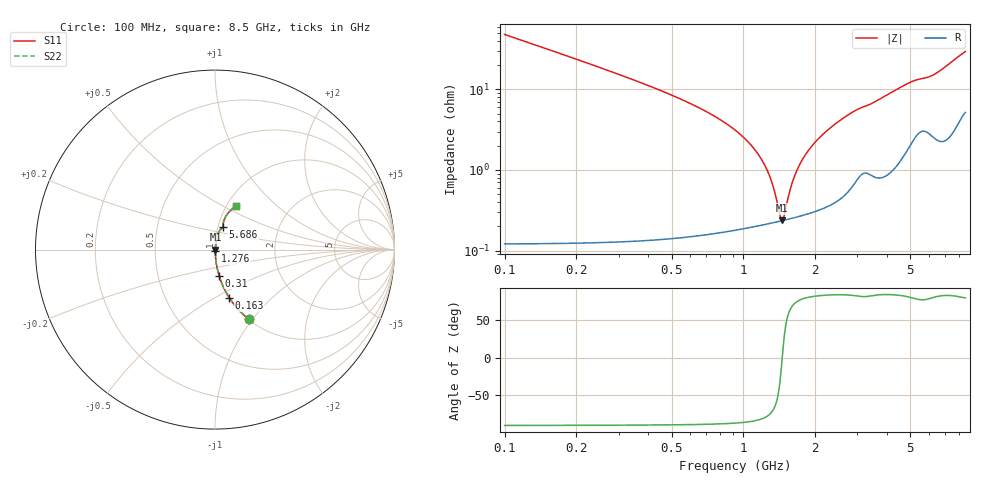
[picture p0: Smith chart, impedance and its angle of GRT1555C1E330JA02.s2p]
!Murata Part Number: GRT1555C1E330JA02
!These Parameters are Measured in Series Mode Connection
!Data Generated on Jun 19, 2026
!  o--ll--o
!Port1  Port2
!  o------o
!Operation Temp=25[degC], DC Bias Voltage=0[V]
!Freq. Start=100[MHz] Stop=9[GHz] 401[Steps]
# Hz S RI R 50
!Freq.(Hz) S11(Real) S11(Imag) S21(Real) S21(Imag) S12(Real) S12(Imag) S22(Real) S22(Imag)
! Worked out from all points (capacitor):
!   401 points, 100 MHz to 8.5 GHz, reference 50 ohm
!   read as one part in series: C = 33 pF near 142 MHz
!   lowest |Z| = 238 mohm at 1.444 GHz (marker M1)
!   series resonance near 1.454 GHz, so ESL is about 360 pH
!   S11 on the Smith chart (normalised r, x): 100 MHz: 1.00, -0.96; 163 MHz: 1.00, -0.58; 310 MHz: 1.00, -0.30; 1.276 GHz: 1.00, -0.02; 5.686 GHz: 1.06, +0.27; 8.5 GHz: 1.10, +0.58
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1e8  0.1879 -0.3893  0.8121 0.3893  0.8121 0.3893  0.1879 -0.3893
1.63e8  0.0796 -0.2686  0.9204 0.2686  0.9204 0.2686  0.0796 -0.2686
3.1e8  0.0228 -0.1449  0.9772 0.1449  0.9772 0.1449  0.0228 -0.1449
5.62e8  0.00672 -0.0724  0.9933 0.0724  0.9933 0.0724  0.00672 -0.0724
1.024e9  0.00245 -0.0237  0.9976 0.0237  0.9976 0.0237  0.00245 -0.0237
1.171e9  0.00225 -0.0144  0.9978 0.0144  0.9978 0.0144  0.00225 -0.0144
1.276e9  0.00222 -0.00867  0.9978 0.00867  0.9978 0.00867  0.00222 -0.00867
1.402e9  0.00229 -0.0024  0.9977 0.0024  0.9977 0.0024  0.00229 -0.0024
1.444e9  0.00233 -0.000437  0.9977 0.000437  0.9977 0.000437  0.00233 -0.000437
1.465e9  0.00236 0.000524  0.9976 -0.000524  0.9976 -0.000524  0.00236 0.000524
1.507e9  0.00241 0.00241  0.9976 -0.00241  0.9976 -0.00241  0.00241 0.00241
1.57e9  0.0025 0.00515  0.9975 -0.00515  0.9975 -0.00515  0.0025 0.00515
1.654e9  0.00265 0.00866  0.9973 -0.00866  0.9973 -0.00866  0.00265 0.00866
1.759e9  0.00287 0.0129  0.9971 -0.0129  0.9971 -0.0129  0.00287 0.0129
1.906e9  0.00325 0.0185  0.9968 -0.0185  0.9968 -0.0185  0.00325 0.0185
2.305e9  0.00469 0.0326  0.9953 -0.0326  0.9953 -0.0326  0.00469 0.0326
2.914e9  0.00948 0.0525  0.9905 -0.0525  0.9905 -0.0525  0.00948 0.0525
4.3e9  0.0192 0.0933  0.9808 -0.0933  0.9808 -0.0933  0.0192 0.0933
5.686e9  0.0455 0.1241  0.9545 -0.1241  0.9545 -0.1241  0.0455 0.1241
5.707e9  0.0456 0.1244  0.9544 -0.1244  0.9544 -0.1244  0.0456 0.1244
7.114e9  0.0578 0.1805  0.9422 -0.1805  0.9422 -0.1805  0.0578 0.1805
8.5e9  0.1165 0.2437  0.8835 -0.2437  0.8835 -0.2437  0.1165 0.2437
